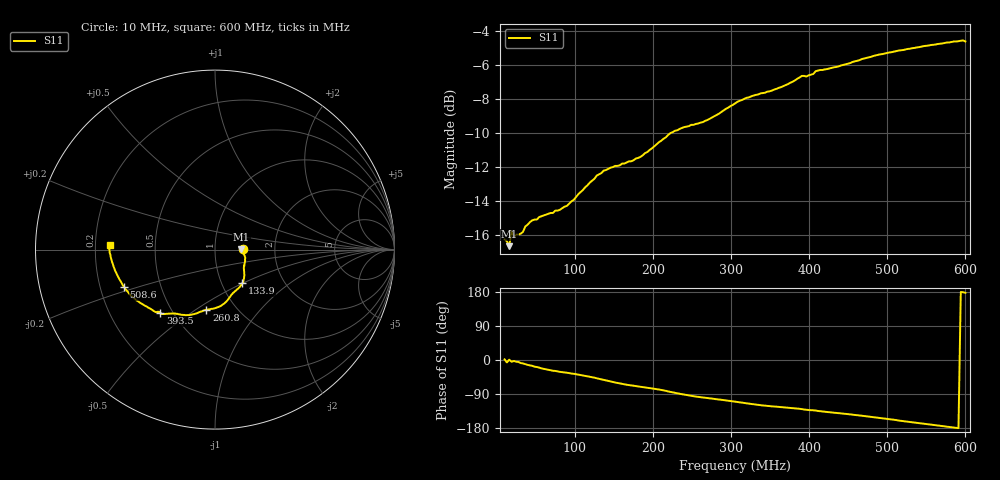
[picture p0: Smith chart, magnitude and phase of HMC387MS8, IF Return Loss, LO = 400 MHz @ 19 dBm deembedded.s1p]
!Hittite Microwave Corporation
!12 Elizabeth Drive
!Chelmsford, MA 01824
!Tel: 978-250-3343
!Fax: 978-250-3373
!Device: HMC387MS8, 450-500 MHz, GaAs MMIC High IP3 Mixer in 8-lead plastic SMT package
!Misc: IF Return Loss, LO = 400 MHz @ 19 dBm, Room
# MHZ S MA R 50
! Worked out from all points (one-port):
!   201 points, 10 MHz to 600 MHz, reference 50 ohm
!   lowest |S11| = -16.7 dB at 15.9 MHz (marker M1), VSWR 1.34, Z = 67.2 + j0.301 ohm
!   |S11| at or under -10 dB: start of sweep to 222.7 MHz
!   S11 on the Smith chart (normalised r, x): 10 MHz: 1.36, +0.01; 133.9 MHz: 1.25, -0.50; 260.8 MHz: 0.73, -0.55; 393.5 MHz: 0.43, -0.39; 508.6 MHz: 0.30, -0.18; 600 MHz: 0.26, +0.02
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10  0.154 1.7
12.95  0.152 -6.4
15.9  0.147 0.9
18.85  0.163 -4.6
21.8  0.156 -2.7
33.6  0.162 -9.1
36.55  0.168 -11.0
45.4  0.175 -15.5
83.75  0.19 -32.0
98.5  0.201 -36.3
113.25  0.219 -41.8
133.9  0.241 -51.0
157.5  0.254 -61.6
184.05  0.269 -70.4
204.7  0.293 -76.8
231.25  0.322 -87.9
260.75  0.339 -98.1
305  0.386 -109.8
337.45  0.413 -119.2
378.75  0.447 -126.9
393.5  0.465 -130.8
408.25  0.48 -133.4
452.5  0.507 -143.4
482  0.532 -150.7
508.55  0.548 -157.8
526.25  0.558 -162.8
576.4  0.583 -176.2
600  0.587 177.4
